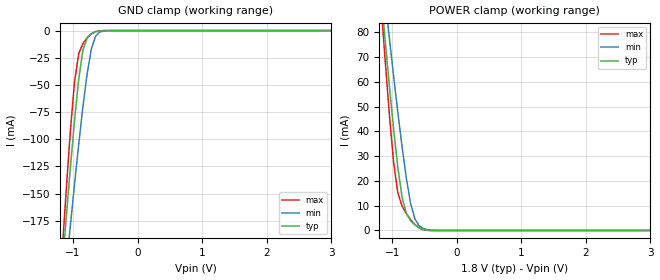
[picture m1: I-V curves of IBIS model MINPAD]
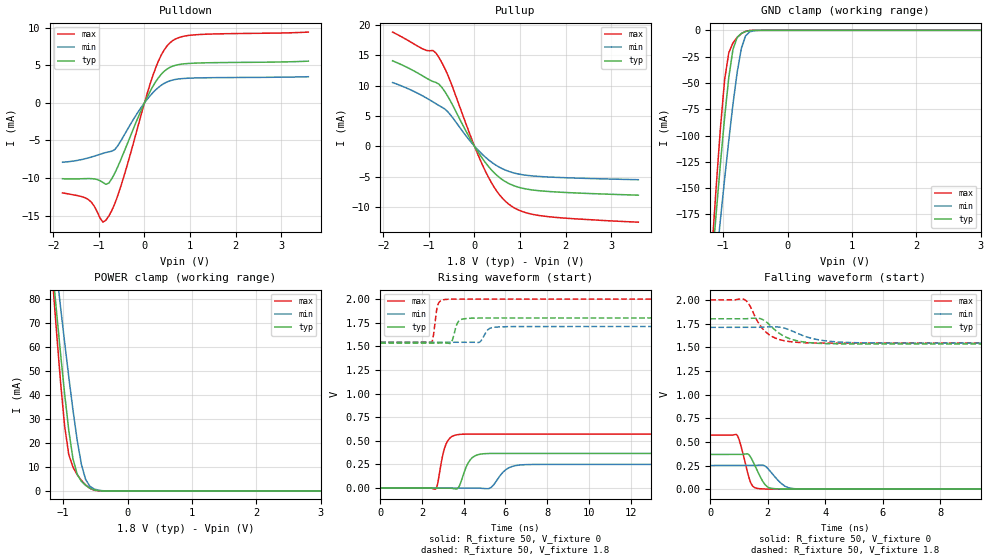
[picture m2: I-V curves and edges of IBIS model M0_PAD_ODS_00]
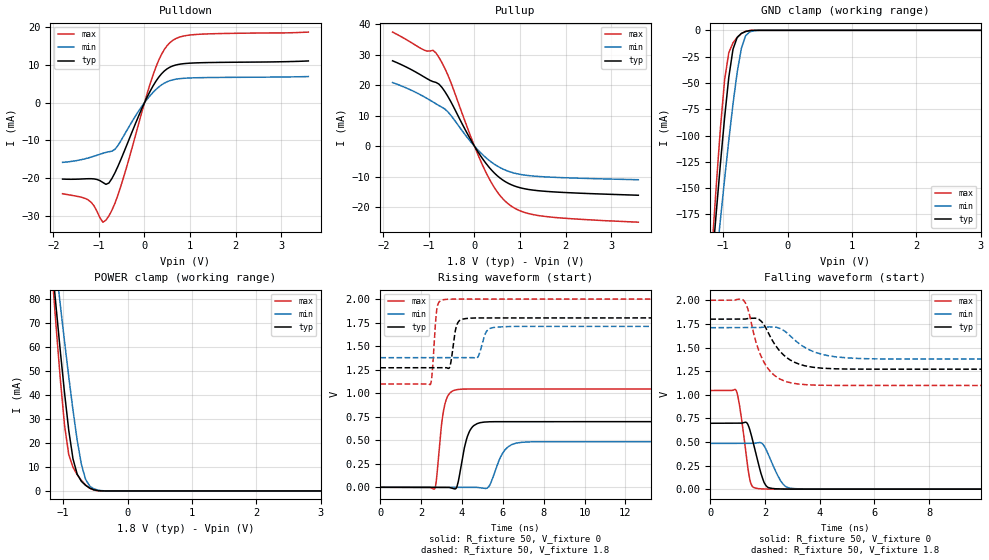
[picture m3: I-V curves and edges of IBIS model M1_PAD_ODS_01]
| Created by SiliconSmart  O-2018.09-SP2-3
[IBIS Ver]   4.0
[File Name]   as31b32bd_1p8_rev1p4.ibs
[File Rev]   1.4
[Date]   Thursday Mar 21 2024
|[Source]   Avalanche Team
|[Notes]   Generated IBIS models from Silicon Smart
|[Rev 1.0]  Initial Release based on extracted netlist
|   Characterization
|[Rev 1.1]  Recharacterization with Hspice, run in high accuracy mode
|[Rev 1.2]  Recharacterization with Hspice, run with parameters inline
|   with the datasheet
|[Rev 1.3]  Recharacterization with Hspice, run with updated VIH/VIL
|   in parallel with datasheet rev X.7
|[Rev 1.4]  Update the pin to the package pinout assignment
|[Disclaimer]   THE MODEL LIBRARIES ARE PROVIDED AS IS.
|[Copyright]   Copyright 2019, Avalanche Technology., All Rights Reserved
[Component]   AS301GB32_BGA
[Manufacturer] Avalanche Technology
| CONTENT :
| This file contains IBIS MODEL for PSRAM device
| AS301GB32
| USAGE :
| The models are derived for the 1.71V to 2.0V I/O Operation.
| Temperatures for model generation: typ: 25, max: -40, min: 125
| Voltages : typ: 1.8V, min: 1.71V, max: 2.0V
| PACKAGES SUPPORTED :
| 142-ball FBGA (15mm x 17mm)
| VERIFICATION
| Errors  : 0
| Warnings: 11
| All warnings due to non-monotonic data:
[Package]
R_pkg   0   0 0
L_pkg   0   0 0
C_pkg   0   0 0
[Pin]   signal_name   model_name   R_pin   L_pin   C_pin
P8   E#   MINPAD   0.254	7.307E-9	1.178E-12
P7   G#   MINPAD   0.243	7.052E-9	1.094E-12
J2   CR#   MINPAD   0.547	10.386E-9	1.789E-12
K3   PG#   MINPAD   0.451	10.329E-9	1.676E-12
M8   W#   MINPAD   0.377	9.020E-9	1.417E-12
M2   ADDR_26   MINPAD   0.425	9.037E-9	1.604E-12
L4   ADDR_25   MINPAD   0.419	9.644E-9	1.527E-12
K13   ADDR_24   MINPAD   0.495	9.978E-9	1.745E-12
M3   ADDR_23   MINPAD   0.371	9.313E-9	1.466E-12
L3   ADDR_22   MINPAD   0.412	9.753E-9	1.540E-12
M7   ADDR_21   MINPAD   0.368	8.765E-9	1.384E-12
P12   ADDR_20   MINPAD   0.287	8.287E-9	1.639E-12
L12   ADDR_19   MINPAD   0.424	10.320E-9	1.620E-12
N11   ADDR_18   MINPAD   0.338	8.691E-9	1.470E-12
N6   ADDR_17   MINPAD   0.309	8.196E-9	1.279E-12
P6   ADDR_16   MINPAD   0.256	7.462E-9	1.204E-12
L13   ADDR_15   MINPAD   0.463	10.719E-9	1.740E-12
M13   ADDR_14   MINPAD   0.421	10.290E-9	1.689E-12
P10   ADDR_13   MINPAD   0.262	7.671E-9	1.349E-12
N10   ADDR_12   MINPAD   0.340	8.540E-9	1.360E-12
M12   ADDR_11   MINPAD   0.402	9.876E-9	1.604E-12
N13   ADDR_10   MINPAD   0.399	9.819E-9	1.696E-12
L11   ADDR_9   MINPAD   0.443	9.732E-9	1.569E-12
M11   ADDR_8   MINPAD   0.436	9.682E-9	1.671E-12
P5   ADDR_7   MINPAD   0.253	7.464E-9	1.277E-12
P3   ADDR_6   MINPAD   0.279	8.031E-9	1.557E-12
N5   ADDR_5   MINPAD   0.313	8.320E-9	1.359E-12
N4   ADDR_4   MINPAD   0.329	8.138E-9	1.428E-12
M4   ADDR_3   MINPAD   0.379	8.543E-9	1.406E-12
N2   ADDR_2   MINPAD   0.378	9.572E-9	1.637E-12
N9   ADDR_1   MINPAD   0.315	8.416E-9	1.305E-12
M9   ADDR_0   MINPAD   0.403	9.225E-9	1.473E-12
E2   DQ_31   MIOPAD   0.365	8.798E-9	1.454E-12
F2   DQ_30   MIOPAD   0.418	9.057E-9	1.576E-12
D2   DQ_29   MIOPAD   0.358	8.697E-9	1.520E-12
E3   DQ_28   MIOPAD   0.348	8.812E-9	1.441E-12
E12   DQ_27   MIOPAD   0.327	8.506E-9	1.443E-12
D10   DQ_26   MIOPAD   0.309	7.715E-9	1.264E-12
C9   DQ_25   MIOPAD   0.279	7.395E-9	1.219E-12
C7   DQ_24   MIOPAD   0.252	6.802E-9	1.108E-12
G4   DQ_23   MIOPAD   0.455	10.071E-9	1.775E-12
G3   DQ_22   MIOPAD   0.457	10.100E-9	1.750E-12
F13   DQ_21   MIOPAD   0.377	9.387E-9	1.566E-12
D13   DQ_20   MIOPAD   0.295	8.231E-9	1.460E-12
C10   DQ_19   MIOPAD   0.293	7.553E-9	1.298E-12
E8   DQ_18   MIOPAD   0.393	8.323E-9	1.436E-12
F6   DQ_17   MIOPAD   0.425	8.913E-9	1.517E-12
E5   DQ_16   MIOPAD   0.379	8.982E-9	1.460E-12
E13   DQ_15   MIOPAD   0.363	8.555E-9	1.474E-12
G11   DQ_14   MIOPAD   0.475	9.536E-9	1.630E-12
E10   DQ_13   MIOPAD   0.404	8.563E-9	1.453E-12
F9   DQ_12   MIOPAD   0.409	9.347E-9	1.513E-12
C8   DQ_11   MIOPAD   0.257	6.782E-9	1.111E-12
C6   DQ_10   MIOPAD   0.238	7.000E-9	1.114E-12
D6   DQ_9   MIOPAD   0.292	7.776E-9	1.248E-12
D4   DQ_8   MIOPAD   0.305	7.782E-9	1.343E-12
G12   DQ_7   MIOPAD   0.502	10.055E-9	1.687E-12
C12   DQ_6   MIOPAD   0.275	7.857E-9	1.346E-12
D11   DQ_5   MIOPAD   0.286	7.835E-9	1.360E-12
D9   DQ_4   MIOPAD   0.306	8.035E-9	1.299E-12
E7   DQ_3   MIOPAD   0.384	8.178E-9	1.375E-12
C5   DQ_2   MIOPAD   0.231	6.786E-9	1.150E-12
D5   DQ_1   MIOPAD   0.307	7.698E-9	1.346E-12
C3   DQ_0   MIOPAD   0.267	7.420E-9	1.241E-12
G13   INT#   MIOPAD   0.480	10.704E-9	1.759E-12
F10   VSSIO   GND   NA   NA   NA
L10   VSSIO   GND   NA   NA   NA
E9   VSSIO   GND   NA   NA   NA
L9   VSSIO   GND   NA   NA   NA
F8   VSSIO   GND   NA   NA   NA
L8   VSSIO   GND   NA   NA   NA
F7   VSSIO   GND   NA   NA   NA
L7   VSSIO   GND   NA   NA   NA
E6   VSSIO   GND   NA   NA   NA
L6   VSSIO   GND   NA   NA   NA
G5   VSSIO   GND   NA   NA   NA
A14   VSS   GND   NA   NA   NA
B14   VSS   GND   NA   NA   NA
C14   VSS   GND   NA   NA   NA
H13   VSS   GND   NA   NA   NA
R14   VSS   GND   NA   NA   NA
T14   VSS   GND   NA   NA   NA
A13   VSS   GND   NA   NA   NA
T13   VSS   GND   NA   NA   NA
A12   VSS   GND   NA   NA   NA
G10   VSS   GND   NA   NA   NA
H10   VSS   GND   NA   NA   NA
J10   VSS   GND   NA   NA   NA
K10   VSS   GND   NA   NA   NA
F5   VSS   GND   NA   NA   NA
L5   VSS   GND   NA   NA   NA
A2   VSS   GND   NA   NA   NA
T2   VSS   GND   NA   NA   NA
A1   VSS   GND   NA   NA   NA
B1   VSS   GND   NA   NA   NA
R1   VSS   GND   NA   NA   NA
T1   VSS   GND   NA   NA   NA
F12   VCCIO   POWER   NA   NA   NA
J12   VCCIO   POWER   NA   NA   NA
E11   VCCIO   POWER   NA   NA   NA
M10   VCCIO   POWER   NA   NA   NA
D8   VCCIO   POWER   NA   NA   NA
N8   VCCIO   POWER   NA   NA   NA
D7   VCCIO   POWER   NA   NA   NA
N7   VCCIO   POWER   NA   NA   NA
M5   VCCIO   POWER   NA   NA   NA
E4   VCCIO   POWER   NA   NA   NA
F3   VCCIO   POWER   NA   NA   NA
J3   VCCIO   POWER   NA   NA   NA
C13   VCC   POWER   NA   NA   NA
P13   VCC   POWER   NA   NA   NA
D12   VCC   POWER   NA   NA   NA
N12   VCC   POWER   NA   NA   NA
C11   VCC   POWER   NA   NA   NA
F11   VCC   POWER   NA   NA   NA
H11   VCC   POWER   NA   NA   NA
J11   VCC   POWER   NA   NA   NA
K11   VCC   POWER   NA   NA   NA
P11   VCC   POWER   NA   NA   NA
C4   VCC   POWER   NA   NA   NA
F4   VCC   POWER   NA   NA   NA
H4   VCC   POWER   NA   NA   NA
J4   VCC   POWER   NA   NA   NA
K4   VCC   POWER   NA   NA   NA
P4   VCC   POWER   NA   NA   NA
D3   VCC   POWER   NA   NA   NA
N3   VCC   POWER   NA   NA   NA
C2   VCC   POWER   NA   NA   NA
P2   VCC   POWER   NA   NA   NA
| IOPAD
[Model Selector] MIOPAD
| Model Description
M0_PAD_ODS_00   ODS_00
M1_PAD_ODS_01   ODS_01
M2_PAD_ODS_10   ODS_10
M3_PAD_ODS_11   ODS_11
| Models and submodels in the file (5): MINPAD (Input), M0_PAD_ODS_00 (I/O), M1_PAD_ODS_01 (I/O), M2_PAD_ODS_10 (I/O), M3_PAD_ODS_11 (I/O)
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[Model] MINPAD
Model_type Input
Enable   Active-High
Vinl  =  0.63
Vinh  =  1.17
| Capacitance  typ   min   max
C_comp   1.624351e-12   1.517192e-12   1.739751e-12
| Variables   typ   min   max
[GND Clamp Reference]   0   0   0
[POWER Clamp Reference]   1.8   1.71   2
[Pulldown Reference]   0   0   0
[Pullup Reference]   1.8   1.71   2
[Temperature Range]   25   125   -40
[Voltage Range]   1.8   1.71   2
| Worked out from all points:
|   GND clamp passes 1 mA (typ) near -0.64 V on its own axis
|   POWER clamp passes 1 mA (typ) near -0.57 V on its own axis
[GND Clamp]
| Voltage   I(typ)   I(min)   I(max)
-1.8V     -720.5mA   -670.5mA   -825.4mA
-1.173V   -222.3mA   -260.3mA   -207.7mA
-1.108V   -173.8mA   -219.8mA   -148.5mA
-1.043V   -127mA     -180.1mA   -93.29mA
-977.6mV  -83.06mA   -141.5mA   -47.18mA
-912.4mV  -44.72mA   -104.6mA   -21.22mA
-847.2mV  -17.98mA   -70.1mA    -11.91mA
-782.1mV  -6.764mA   -39.85mA   -6.651mA
-716.9mV  -2.937mA   -17.13mA   -3.044mA
-651.7mV  -1.118mA   -5.25mA    -949.8uA
-456.2mV  -3.975uA   -74.4uA    -419.6nA
3.6V      0A         0A         0A
[POWER Clamp]
| Voltage   I(typ)   I(min)   I(max)
-1.8V     287.1mA    268.3mA    329.6mA
-1.173V   94.89mA    108.5mA    91.02mA
-1.108V   76.1mA     92.66mA    67.97mA
-1.043V   57.9mA     77.16mA    46.14mA
-977.6mV  40.62mA    62.05mA    27.14mA
-912.4mV  25.13mA    47.46mA    15.06mA
-847.2mV  13.38mA    33.64mA    9.853mA
-716.9mV  4.014mA    11.09mA    4.394mA
-651.7mV  2.34mA     4.821mA    2.483mA
-586.6mV  1.18mA     2.003mA    1.113mA
-325.9mV  1.153uA    19.85uA    110.1nA
3.6V      0A         0A         0A
[Model] M0_PAD_ODS_00
Model_type I/O
Enable   Active-High
Vinl  =  0.63
Vinh  =  1.17
Vmeas =  0.9
Cref  =  30e-12
| Capacitance  typ   min   max
C_comp   1.627116e-12   1.521588e-12   1.744735e-12
| Variables   typ   min   max
[GND Clamp Reference]   0   0   0
[POWER Clamp Reference]   1.8   1.71   2
[Pulldown Reference]   0   0   0
[Pullup Reference]   1.8   1.71   2
[Temperature Range]   25   125   -40
[Voltage Range]   1.8   1.71   2
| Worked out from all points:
|   slope of the pulldown table from 0 to 0.27 V, typ, clamps not added: 89.8 ohm
|   slope of the pullup table from 0 to 0.27 V, typ, clamps not added: 90.4 ohm
|   GND clamp passes 1 mA (typ) near -0.64 V on its own axis
|   POWER clamp passes 1 mA (typ) near -0.57 V on its own axis
|   falling waveform, R_fixture 50, V_fixture 0: 20-80 % time 364ps typ, 459ps min, 289ps max; typ from 0.367 V to 0 V
|   falling waveform, R_fixture 50, V_fixture 1.8: 20-80 % time 770ps typ, 991ps min, 610ps max; typ from 1.8 V to 1.53 V
|   rising waveform, R_fixture 50, V_fixture 0: 20-80 % time 416ps typ, 570ps min, 332ps max; typ from 0 V to 0.367 V
|   rising waveform, R_fixture 50, V_fixture 1.8: 20-80 % time 213ps typ, 281ps min, 164ps max; typ from 1.53 V to 1.8 V
[GND Clamp]
| Voltage   I(typ)   I(min)   I(max)
-1.8V     -720.5mA   -670.5mA   -825.4mA
-1.173V   -222.3mA   -260.3mA   -207.7mA
-1.108V   -173.8mA   -219.8mA   -148.5mA
-1.043V   -127mA     -180.1mA   -93.3mA
-977.6mV  -83.06mA   -141.5mA   -47.19mA
-912.4mV  -44.72mA   -104.6mA   -21.23mA
-847.2mV  -17.99mA   -70.1mA    -11.92mA
-782.1mV  -6.766mA   -39.85mA   -6.657mA
-716.9mV  -2.938mA   -17.13mA   -3.048mA
-651.7mV  -1.119mA   -5.25mA    -952uA
-456.2mV  -3.98uA    -74.41uA   -422.2nA
3.6V      0A         0A         0A
[POWER Clamp]
| Voltage   I(typ)   I(min)   I(max)
-1.8V     287.1mA    268.3mA    329.6mA
-1.173V   94.89mA    108.5mA    91.02mA
-1.108V   76.1mA     92.66mA    67.97mA
-1.043V   57.9mA     77.16mA    46.14mA
-977.6mV  40.62mA    62.05mA    27.14mA
-912.4mV  25.13mA    47.46mA    15.06mA
-847.2mV  13.38mA    33.64mA    9.853mA
-716.9mV  4.014mA    11.09mA    4.394mA
-651.7mV  2.34mA     4.821mA    2.483mA
-586.6mV  1.18mA     2.003mA    1.113mA
-325.9mV  1.153uA    19.85uA    110.1nA
3.6V      0A         0A         0A
[Pulldown]
| Voltage   I(typ)   I(min)   I(max)
-1.8V     -10.09mA   -7.898mA   -11.97mA
-1.238V   -10.07mA   -7.328mA   -12.83mA
-912.4mV  -10.59mA   -6.717mA   -15.86mA
-847.2mV  -10.83mA   -6.605mA   -15.6mA
-716.9mV  -10.08mA   -6.431mA   -14.3mA
-521.4mV  -7.575mA   -5.077mA   -11.12mA
-65.17mV  -872uA     -545.4uA   -1.404mA
248.3mV   2.817mA    1.73mA     4.683mA
434.5mV   4.193mA    2.586mA    7.041mA
620.7mV   4.869mA    3.026mA    8.258mA
1.179V    5.284mA    3.307mA    9.058mA
3.6V      5.531mA    3.462mA    9.391mA
[Pullup]
| Voltage   I(typ)   I(min)   I(max)
-1.8V     14.07mA    10.49mA    18.8mA
-1.108V   11.45mA    8.161mA    15.93mA
-912.4mV  10.66mA    7.301mA    15.78mA
-782.1mV  10.22mA    6.706mA    14.62mA
-586.6mV  8.214mA    5.673mA    11.74mA
-65.17mV  835.7uA    571.5uA    1.251mA
248.3mV   -2.782mA   -1.866mA   -4.251mA
496.6mV   -4.831mA   -3.242mA   -7.473mA
744.8mV   -6.111mA   -4.126mA   -9.499mA
1.055V    -6.927mA   -4.698mA   -10.78mA
1.428V    -7.337mA   -4.986mA   -11.42mA
3.6V      -8.069mA   -5.52mA    -12.52mA
[Ramp]
dV/dt_r   0.220223/0.415702n  0.150081/0.569672n  0.34276/0.331988n
dV/dt_f   0.159898/0.770039n  0.100158/0.991323n  0.274318/0.609698n
R_load = 50
[Falling Waveform]
R_fixture = 50
V_fixture = 0
V_fixture_min = 0
V_fixture_max = 0
| Time   V(typ)   V(min)   V(max)
0s        367mV      250.1mV    571.3mV
923.8ps   367.3mV    250.7mV    573.7mV
1.037ns   367.3mV    250.7mV    489.3mV
1.291ns   372.9mV    250.9mV    184mV
1.42ns    330.5mV    250.9mV    60.14mV
1.744ns   128.3mV    254.8mV    4.316mV
2.055ns   13.67mV    200.4mV    1.169mV
2.601ns   1.34mV     30.95mV    220.5uV
2.98ns    480.5uV    4.171mV    216.1uV
21.88ns   3.869uV    78.26nV    -3.43uV
[Falling Waveform]
R_fixture = 50
V_fixture = 1.8
V_fixture_min = 1.71
V_fixture_max = 2
| Time   V(typ)   V(min)   V(max)
0s        1.8V       1.71V      2V
1.194ns   1.801V     1.71V      2.003V
1.367ns   1.805V     1.71V      1.943V
1.68ns    1.806V     1.711V     1.755V
1.949ns   1.766V     1.714V     1.656V
2.444ns   1.638V     1.711V     1.578V
2.887ns   1.578V     1.666V     1.554V
3.81ns    1.541V     1.576V     1.544V
5.079ns   1.534V     1.547V     1.543V
21.88ns   1.534V     1.543V     1.543V
[Rising Waveform]
R_fixture = 50
V_fixture = 0
V_fixture_min = 0
V_fixture_max = 0
| Time   V(typ)   V(min)   V(max)
0s        3.036nV    85.33nV    -62.8nV
2.644ns   -691.4uV   -545.1uV   -11.75mV
3.145ns   -822.4uV   -648.4uV   462.5mV
3.72ns    -1.25mV    -766.9uV   565.8mV
4.314ns   300mV      -889.5uV   570.7mV
5.019ns   364.1mV    -5.657mV   570.7mV
5.313ns   366.1mV    6.668mV    570.7mV
6.157ns   366.1mV    214mV      570.8mV
6.888ns   366.1mV    247mV      570.8mV
21.88ns   367mV      250.1mV    571.3mV
[Rising Waveform]
R_fixture = 50
V_fixture = 1.8
V_fixture_min = 1.71
V_fixture_max = 2
| Time   V(typ)   V(min)   V(max)
0s        1.534V     1.543V     1.543V
2.445ns   1.534V     1.543V     1.54V
2.53ns    1.534V     1.543V     1.594V
2.745ns   1.534V     1.543V     1.929V
3.139ns   1.534V     1.543V     1.996V
3.396ns   1.538V     1.543V     1.999V
3.757ns   1.766V     1.543V     1.999V
4.265ns   1.797V     1.543V     1.999V
5.688ns   1.8V       1.705V     1.999V
21.88ns   1.8V       1.71V      2V
[Model] M1_PAD_ODS_01
Model_type I/O
Enable   Active-High
Vinl  =  0.63
Vinh  =  1.17
Vmeas =  0.9
Cref  =  30e-12
| Capacitance  typ   min   max
C_comp   1.627116e-12   1.521588e-12   1.744735e-12
| Variables   typ   min   max
[GND Clamp Reference]   0   0   0
[POWER Clamp Reference]   1.8   1.71   2
[Pulldown Reference]   0   0   0
[Pullup Reference]   1.8   1.71   2
[Temperature Range]   25   125   -40
[Voltage Range]   1.8   1.71   2
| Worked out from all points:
|   slope of the pulldown table from 0 to 0.27 V, typ, clamps not added: 44.9 ohm
|   slope of the pullup table from 0 to 0.27 V, typ, clamps not added: 45.3 ohm
|   GND clamp passes 1 mA (typ) near -0.64 V on its own axis
|   POWER clamp passes 1 mA (typ) near -0.57 V on its own axis
|   falling waveform, R_fixture 50, V_fixture 0: 20-80 % time 370ps typ, 463ps min, 286ps max; typ from 0.698 V to 0 V
|   falling waveform, R_fixture 50, V_fixture 1.8: 20-80 % time 821ps typ, 1.04ns min, 652ps max; typ from 1.8 V to 1.27 V
|   rising waveform, R_fixture 50, V_fixture 0: 20-80 % time 411ps typ, 571ps min, 311ps max; typ from 0 V to 0.698 V
|   rising waveform, R_fixture 50, V_fixture 1.8: 20-80 % time 216ps typ, 282ps min, 166ps max; typ from 1.27 V to 1.8 V
[GND Clamp]
| Voltage   I(typ)   I(min)   I(max)
-1.8V     -720.5mA   -670.5mA   -825.4mA
-1.173V   -222.3mA   -260.3mA   -207.7mA
-1.108V   -173.8mA   -219.8mA   -148.5mA
-1.043V   -127mA     -180.1mA   -93.3mA
-977.6mV  -83.06mA   -141.5mA   -47.19mA
-912.4mV  -44.72mA   -104.6mA   -21.23mA
-847.2mV  -17.99mA   -70.1mA    -11.92mA
-782.1mV  -6.766mA   -39.85mA   -6.657mA
-716.9mV  -2.938mA   -17.13mA   -3.048mA
-651.7mV  -1.119mA   -5.25mA    -952uA
-456.2mV  -3.98uA    -74.41uA   -422.2nA
3.6V      0A         0A         0A
[POWER Clamp]
| Voltage   I(typ)   I(min)   I(max)
-1.8V     287.1mA    268.3mA    329.6mA
-1.173V   94.89mA    108.5mA    91.02mA
-1.108V   76.1mA     92.66mA    67.97mA
-1.043V   57.9mA     77.16mA    46.14mA
-977.6mV  40.62mA    62.05mA    27.14mA
-912.4mV  25.13mA    47.46mA    15.06mA
-847.2mV  13.38mA    33.64mA    9.853mA
-716.9mV  4.014mA    11.09mA    4.394mA
-651.7mV  2.34mA     4.821mA    2.483mA
-586.6mV  1.18mA     2.003mA    1.113mA
-325.9mV  1.153uA    19.85uA    110.1nA
3.6V      0A         0A         0A
[Pulldown]
| Voltage   I(typ)   I(min)   I(max)
-1.8V     -20.26mA   -15.83mA   -24.15mA
-1.238V   -20.17mA   -14.67mA   -25.78mA
-912.4mV  -21.17mA   -13.42mA   -31.69mA
-847.2mV  -21.66mA   -13.2mA    -31.16mA
-716.9mV  -20.14mA   -12.86mA   -28.56mA
-521.4mV  -15.14mA   -10.15mA   -22.2mA
-65.17mV  -1.742mA   -1.091mA   -2.802mA
248.3mV   5.63mA     3.46mA     9.353mA
434.5mV   8.383mA    5.171mA    14.07mA
620.7mV   9.735mA    6.051mA    16.51mA
1.179V    10.57mA    6.614mA    18.12mA
3.6V      11.06mA    6.923mA    18.71mA
[Pullup]
| Voltage   I(typ)   I(min)   I(max)
-1.8V     28.03mA    20.89mA    37.45mA
-1.108V   22.74mA    16.24mA    31.55mA
-912.4mV  21.2mA     14.52mA    31.47mA
-782.1mV  20.39mA    13.35mA    29.17mA
-521.4mV  14.66mA    10.17mA    21.02mA
-130.3mV  3.403mA    2.332mA    5.058mA
186.2mV   -4.285mA   -2.877mA   -6.521mA
496.6mV   -9.629mA   -6.461mA   -14.9mA
744.8mV   -12.18mA   -8.22mA    -18.94mA
1.055V    -13.81mA   -9.36mA    -21.49mA
1.49V     -14.71mA   -9.993mA   -22.92mA
3.6V      -16.07mA   -10.99mA   -24.92mA
[Ramp]
dV/dt_r   0.418626/0.410816n  0.290552/0.571412n  0.626829/0.311374n
dV/dt_f   0.317973/0.820722n  0.199636/1.04338n  0.541445/0.651669n
R_load = 50
[Falling Waveform]
R_fixture = 50
V_fixture = 0
V_fixture_min = 0
V_fixture_max = 0
| Time   V(typ)   V(min)   V(max)
0s        697.7mV    484.3mV    1.045V
951.4ps   698.1mV    484.5mV    1.042V
1.108ns   698.1mV    484.5mV    814.4mV
1.331ns   703.6mV    484.6mV    322mV
1.452ns   622mV      484.6mV    93.29mV
1.73ns    303.2mV    490.6mV    6.618mV
2.068ns   27.7mV     403mV      1.399mV
2.572ns   2.158mV    87.65mV    450.6uV
3.037ns   658.8uV    6.568mV    439.8uV
21.88ns   1.498nV    129.2nV    255.6nV
[Falling Waveform]
R_fixture = 50
V_fixture = 1.8
V_fixture_min = 1.71
V_fixture_max = 2
| Time   V(typ)   V(min)   V(max)
0s        1.8V       1.71V      2V
1.215ns   1.801V     1.71V      2V
1.378ns   1.807V     1.71V      1.904V
1.7ns     1.808V     1.71V      1.529V
1.992ns   1.728V     1.717V     1.329V
2.553ns   1.458V     1.701V     1.165V
3.071ns   1.345V     1.583V     1.119V
4.039ns   1.282V     1.431V     1.1V
5.423ns   1.271V     1.384V     1.098V
21.88ns   1.27V      1.377V     1.098V
[Rising Waveform]
R_fixture = 50
V_fixture = 0
V_fixture_min = 0
V_fixture_max = 0
| Time   V(typ)   V(min)   V(max)
0s        2.474nV    66.45nV    166.5nV
2.668ns   -425.3uV   -220uV     -14.74mV
3.141ns   -500.7uV   -259uV     861mV
3.645ns   -17.16mV   -300.5uV   1.033V
4.267ns   540.5mV    -351.8uV   1.044V
4.874ns   685.9mV    -4.978mV   1.044V
5.31ns    695.8mV    6.141mV    1.044V
6.12ns    697mV      401.5mV    1.044V
6.901ns   697.1mV    477.2mV    1.044V
21.88ns   697.7mV    484.3mV    1.045V
[Rising Waveform]
R_fixture = 50
V_fixture = 1.8
V_fixture_min = 1.71
V_fixture_max = 2
| Time   V(typ)   V(min)   V(max)
0s        1.27V      1.377V     1.098V
2.449ns   1.271V     1.378V     1.092V
2.769ns   1.271V     1.378V     1.892V
3.098ns   1.271V     1.378V     1.993V
3.393ns   1.274V     1.378V     1.999V
3.717ns   1.703V     1.378V     2V
4.17ns    1.792V     1.378V     2V
4.743ns   1.799V     1.375V     2V
5.693ns   1.799V     1.701V     2V
21.88ns   1.8V       1.71V      2V
